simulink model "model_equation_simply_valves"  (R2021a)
settings: Solver=FixedStepAuto  StartTime=0.0  StopTime=10.0  FixedStep=Ts  RelTol=1e-3
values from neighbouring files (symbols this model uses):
  acc_bm = 1e-2    (= 0.01)    [params.m]
  acc_C = -1/g    (= -0.101936799185)    [params.m]
  acc_enable = 1    [params.m]
  acc_km = 1e-1    (= 0.1)    [params.m]
  acc_noise_var = 1e-2    (= 0.01)    [params.m]
  air_leak = 1    [ensemble_generate_from_model.m]    (also in params.m = 0)
  B_hs = 1e2    (= 100)    [params.m]
  b_large_bot = 1400    [params.m]
  b_large_up = 1400    [params.m]
  b_small_bot = 1082.6    [params.m]    (also in load_fault_code_params.m)
  b_small_up = 1543.1    [params.m]    (also in load_fault_code_params.m)
  bot_damp_start = 0.01054    [params.m]
  C_1 = sqrt(gamma/R*(2/(gamma+1))^((gamma+1)/(gamma-1)))    [params.m]
  C_2 = sqrt((2*gamma)/(R*(gamma-1)))    [params.m]
  C_A_in = 6.8608e-07    [params.m]    (also in load_fault_code_params.m)
  C_A_out = 5.2299e-07    [params.m]    (also in load_fault_code_params.m)
  C_B_in = 1.8721e-07    [params.m]    (also in load_fault_code_params.m)
  C_B_out = 9.8141e-07    [params.m]    (also in load_fault_code_params.m)
  C_leak = 1e-15    [params.m]
  counter_bits = 32    [params.m]
  cycle = 0    [params.m]    (also in ensemble_process.m = data.Cycle{1,1}.Data)
  F_c = 0    [params.m]
  F_df = 0    [params.m]
  F_sf = 0    [params.m]
  flow_C = flow_enable/flow_C_ratio/conv_SI    (= 59999.988)    [params.m]
  flow_C_ratio = dm_max/U_f_max    (= 1)    [params.m]
  flow_noise_var = 1e-6    (= 1e-06)    [params.m]
  flow_noise_var_con = 1e-6    (= 1e-06)    [params.m]
  flow_offset_con = 0    [params.m]
  flow_offset_ex = 0    [params.m]
  g = 9.81    [params.m]    (also in Conversion_Acc.m)
  gamma = 1.4    [params.m]
  gn = 0    [params.m]
  gp = 0.19382    [params.m]
  id = 0    [params.m]
  K_hs = 1e7    (= 10000000)    [params.m]
  k_small_bot = 0    [params.m]
  k_small_up = 0    [params.m]
  L = 0.2    [params.m]    (also in hammerstein_wiener_model_estimation.m = NaN(N,nk))
  LargeDamper_bottom = member.LargeDamper_bottom{1,1}.Variables    [identification_faultcode.m]    (also in params.m = 0; config_print.m; models_compire.m)
  LargeDamper_upper = member.LargeDamper_upper{1,1}.Variables    [identification_faultcode.m]    (also in params.m = 0; config_print.m; models_compire.m)
  M = 6.7798462575453    (= 6.77984625755)    [params.m]
  M_L = member.("Settings.Load"){1,1}{1,1}    [identification_faultcode.m]    (also in params.m = 6.25; config_print.m; models_compire.m)
  P_0 = 101325    [params.m]
  p_A0 = P_0    (= 101325)    [params.m]
  p_B0 = P_s    (= 600000)    [params.m]
  P_cr = 0.20105    [params.m]    (also in load_fault_code_params.m)
  P_cr_ref = P_cr    (= 0.528281787717)    [params.m]
  P_s = 6e5    (= 600000)    [params.m]
  prox_bot_band = 4e-4    (= 0.0004)    [params.m]
  prox_up_band = 0.1925    [params.m]
  R = 287.1    [params.m]
  resolution = 7.8125e-6    (= 7.8125e-06)    [params.m]    (also in filtering.m; Conversion_Enc.m; pokus.m)
  S_0 = S_A-S_B    (= 5.02654824574e-05)    [params.m]
  S_A = (pi*d_A^2)/4    (= 0.000314159265359)    [params.m]
  S_B = S_A-(pi*d_S^2)/4    (= 0.000263893782902)    [params.m]
  sg_C = Us/F_max    (= 0.005)    [params.m]
  sg_enable = 1    [params.m]
  sg_noise_var = 1e-1    (= 0.1)    [params.m]
  SmallDamper_bottom = member.SmallDamper_bottom{1,1}.Variables    [identification_faultcode.m]    (also in params.m = 6; config_print.m; models_compire.m)
  SmallDamper_upper = member.SmallDamper_upper{1,1}.Variables    [identification_faultcode.m]    (also in params.m = 4; config_print.m; models_compire.m)
  spool_dynamic = 0.02116    [params.m]
  spool_valve_time_delay = 0.01    [params.m]
  T = 281.7    [params.m]    (also in identification_nn.m = cell2mat(T); nn_using.m = tonndata(mimo_T,false,false); nn.m = T(3:end); data_parser.m = T(3:end))
  threshold = 2^(counter_bits - 1)    (= 2147483648)    [params.m]
  Ts = 1/Freq    (= 0.001)    [params.m]    (also in hammerstein_wiener_model_estimation.m; extract_signals_from_member.m; models_compire.m)
  up_damp_start = 0.18123    [params.m]
  V_0A = S_A*0.015    (= 4.71238898038e-06)    [params.m]
  V_0B = S_B*0.015    (= 3.95840674352e-06)    [params.m]
libraries: eeQuadratureDecoder x1

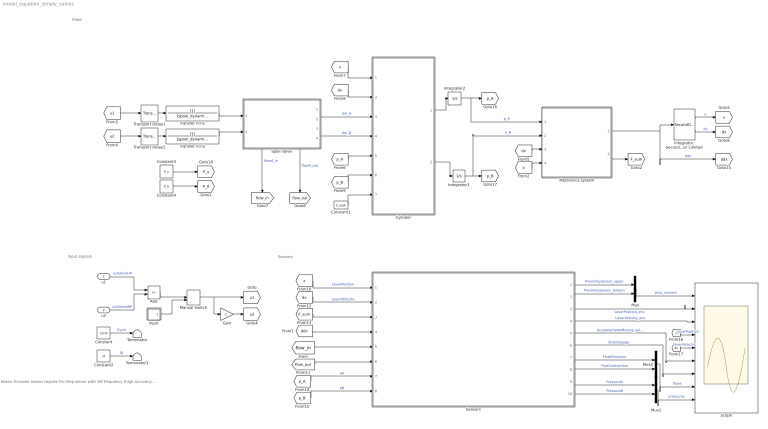
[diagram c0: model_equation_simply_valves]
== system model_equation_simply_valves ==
  note: Sensors
  note: Notes: Encoder sensor require Fix-Step solver with 1M frequency (high accuracy of sensor). For faster-simulation Ts = 1e-3.
  note: Plant
  note: Input signals
  u1 : Inport
  u2 : Inport  Port=2
  Add : Sum  Inputs=-+
  Constant : Constant  Value=cycle  OutDataTypeStr=double
  Constant1 : Constant  Value=C_leak
  Constant2 : Constant  Value=id  OutDataTypeStr=double
  Constant3 : Constant  Value=P_s
  Constant4 : Constant  Value=P_0
  Cylinder : MATLAB Function  TreatAsAtomicUnit=on
  Gain : Gain  Gain=-1
  "Integrator, Second-Order Limited" : SecondOrderIntegrator  ICX=x0  UpperLimitX=gp  LowerLimitX=gn
  Integrator2 : Integrator  InitialCondition=p_A0
  Integrator3 : Integrator  InitialCondition=p_B0
  Manual Switch : ManualSwitch  CurrentSetting=0
  Mechanica system : MATLAB Function  TreatAsAtomicUnit=on
  Mux : Mux  Inputs=2
  Mux1 : Mux  Inputs=2
  Mux2 : Mux  Inputs=2
  Scope : Scope  NumInputPorts=9
  Sensors : Subsystem
  Spoll valve : Subsystem
  Terminator : Terminator
  Terminator1 : Terminator
  Transfer Fcn1 : TransferFcn  Denominator=[spool_dynamic 1]
  Transfer Fcn2 : TransferFcn  Denominator=[spool_dynamic 1]
  Transport Delay1 : TransportDelay  DelayTime=spool_valve_time_delay
  Transport Delay2 : TransportDelay  DelayTime=spool_valve_time_delay
  input : Subsystem
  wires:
  Sensors/3(encoder_LeverPosition) -> Scope/2  "LeverPosition_enc"
  [ddx] -> Sensors/4(ddx)
  input/1(Out1) -> Manual Switch/2
  Sensors/8(FlowContraction) -> Mux2/2  "FlowContraction"
  Mechanica system/1(ddx) -> [ddx], "Integrator, Second-Order Limited"/1  "ddx"
  Constant3/1 -> [P_s]
  [dx] -> Sensors/2(LeverVelocity)  "LeverVelocity"
  [p_B] -> Sensors/8(pB)  "pB"
  u1/1 -> Add/1  "outValveHP"
  Integrator2/1 -> [p_A], Mechanica system/1(p_A)  "p_A"
  Add/1 -> Manual Switch/1
  Mux2/1 -> Scope/8  "flows"
  Transport Delay2/1 -> Transfer Fcn2/1
  Manual Switch/1 -> Gain/1, [u1]
  Sensors/1(ProximitySensor_upper) -> Mux/1  "ProximitySensor_upper"
  "Integrator, Second-Order Limited"/2 -> [dx]  "dx"
  Transfer Fcn1/1 -> Spoll valve/1(u_A)
  Spoll valve/4(flow_out) -> [flow_out]  "flowA_out"
  [flow_in] -> Sensors/5(dm_A_in)
  Transfer Fcn2/1 -> Spoll valve/2(u_B1)
  [F_sum] -> Sensors/3(F)
  [dx] -> Mechanica system/3(dx)
  [u1] -> Transport Delay1/1
  Sensors/2(ProximitySensor_bottom) -> Mux/2  "ProximitySensor_bottom"
  [p_B] -> Cylinder/6(p_B)
  Sensors/4(encoder_LeverVelocity) -> Scope/3  "LeverVelocity_enc"
  Spoll valve/1(dm_A) -> Cylinder/3(dm_A)  "dm_A"
  Spoll valve/3(flow_in) -> [flow_in]  "flowA_in"
  Sensors/7(FlowExtrusion) -> Mux2/1  "FlowExtrusion"
  [x] -> Cylinder/1(x)
  u2/1 -> Add/2  "outValveWP"
  [p_A] -> Cylinder/5(p_A)
  [dx] -> Scope/5  "LeverVelocity"
  [x] -> Sensors/1(LeverPosition)  "LeverPosition"
  [p_A] -> Sensors/7(pA)  "pA"
  Sensors/9(PressureA) -> Mux1/1  "PressureA"
  Spoll valve/2(dm_B) -> Cylinder/4(dm_B)  "dm_B"
  Transport Delay1/1 -> Transfer Fcn1/1
  "Integrator, Second-Order Limited"/1 -> [x]  "x"
  Sensors/5(AccelerometerMoving axisZ) -> Scope/6  "AccelerometerMoving_axisZ"
  [dx] -> Cylinder/2(dx)
  Mechanica system/2(F_sum_strain) -> [F_sum]
  Mux/1 -> Scope/1  "prox_sensors"
  [flow_out] -> Sensors/6(dm_A_out)
  Sensors/6(StrainGauge) -> Scope/7  "StrainGauge"
  Mux1/1 -> Scope/9  "pressures"
  Gain/1 -> [u2]
  [x] -> Scope/4  "LeverPosition"
  [u2] -> Transport Delay2/1
  Constant/1 -> Terminator/1  "Cycle"
  Sensors/10(PressureB) -> Mux1/2  "PressureB"
  Cylinder/1(dp_A) -> Integrator2/1
  Constant1/1 -> Cylinder/7(C_leak)
  [x] -> Mechanica system/4(x)
  Constant4/1 -> [P_0]
  Integrator3/1 -> Mechanica system/2(p_B), [p_B]  "p_B"
  Cylinder/2(dp_B) -> Integrator3/1
  Constant2/1 -> Terminator1/1  "ID"

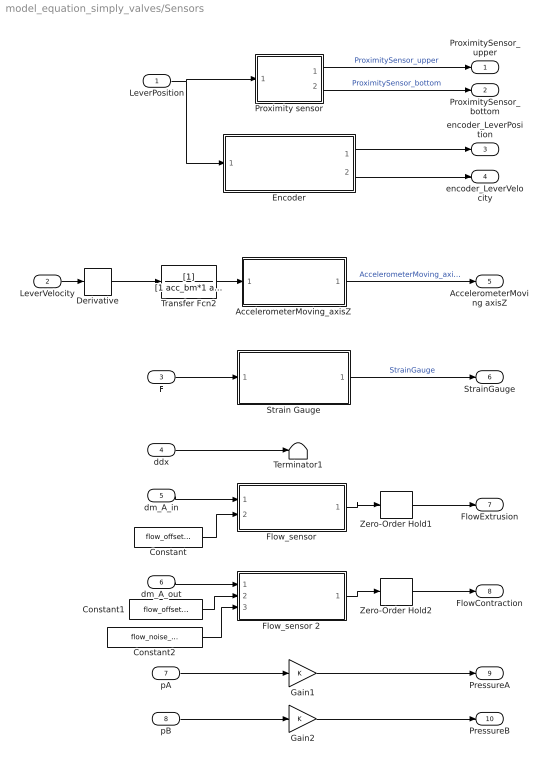
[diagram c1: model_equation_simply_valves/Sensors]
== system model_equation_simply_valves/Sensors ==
  LeverPosition : Inport
  LeverVelocity : Inport  Port=2
  F : Inport  Port=3
  ddx : Inport  Port=4
  dm_A_in : Inport  Port=5
  dm_A_out : Inport  Port=6
  pA : Inport  Port=7
  pB : Inport  Port=8
  AccelerometerMoving_axisZ : MATLAB Function  TreatAsAtomicUnit=on
  Constant : Constant  Value=flow_offset_ex
  Constant1 : Constant  Value=flow_offset_con
  Constant2 : Constant  Value=flow_noise_var_con
  Derivative : Derivative
  Encoder : Subsystem
  Flow_sensor : MATLAB Function  TreatAsAtomicUnit=on
  Flow_sensor 2 : MATLAB Function  TreatAsAtomicUnit=on
  Gain1 : Gain
  Gain2 : Gain
  Proximity sensor : MATLAB Function  TreatAsAtomicUnit=on
  Strain Gauge : MATLAB Function  TreatAsAtomicUnit=on
  Terminator1 : Terminator
  Transfer Fcn2 : TransferFcn  Denominator=[1 acc_bm*1 acc_km*1]
  Zero-Order Hold1 : ZeroOrderHold  SampleTime=Ts
  Zero-Order Hold2 : ZeroOrderHold  SampleTime=Ts
  ProximitySensor_upper : Outport
  ProximitySensor_bottom : Outport  Port=2
  encoder_LeverPosition : Outport  Port=3
  encoder_LeverVelocity : Outport  Port=4
  AccelerometerMoving axisZ : Outport  Port=5
  StrainGauge : Outport  Port=6
  FlowExtrusion : Outport  Port=7
  FlowContraction : Outport  Port=8
  PressureA : Outport  Port=9
  PressureB : Outport  Port=10
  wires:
  F/1 -> Strain Gauge/1(F)
  dm_A_out/1 -> Flow_sensor 2/1(dm_A)
  pB/1 -> Gain2/1
  Flow_sensor/1(dm_A_sensor) -> Zero-Order Hold1/1
  ddx/1 -> Terminator1/1
  AccelerometerMoving_axisZ/1(acc_measured) -> AccelerometerMoving axisZ/1  "AccelerometerMoving_axisZ"
  Encoder/1(encoder_LeverPosition) -> encoder_LeverPosition/1
  Gain2/1 -> PressureB/1
  Proximity sensor/1(up) -> ProximitySensor_upper/1  "ProximitySensor_upper"
  LeverVelocity/1 -> Derivative/1
  Strain Gauge/1(F_measured) -> StrainGauge/1  "StrainGauge"
  Flow_sensor 2/1(dm_A_sensor) -> Zero-Order Hold2/1
  Proximity sensor/2(bot) -> ProximitySensor_bottom/1  "ProximitySensor_bottom"
  Zero-Order Hold2/1 -> FlowContraction/1
  pA/1 -> Gain1/1
  dm_A_in/1 -> Flow_sensor/1(dm_A)
  Zero-Order Hold1/1 -> FlowExtrusion/1
  LeverPosition/1 -> Encoder/1(x), Proximity sensor/1(x)
  Gain1/1 -> PressureA/1
  Encoder/2(encoder_LeverVelocity) -> encoder_LeverVelocity/1
  Constant/1 -> Flow_sensor/2(flow_offset)
  Constant1/1 -> Flow_sensor 2/2(flow_offset)
  Constant2/1 -> Flow_sensor 2/3(flow_noise_var)
  Derivative/1 -> Transfer Fcn2/1
  Transfer Fcn2/1 -> AccelerometerMoving_axisZ/1(ddx)

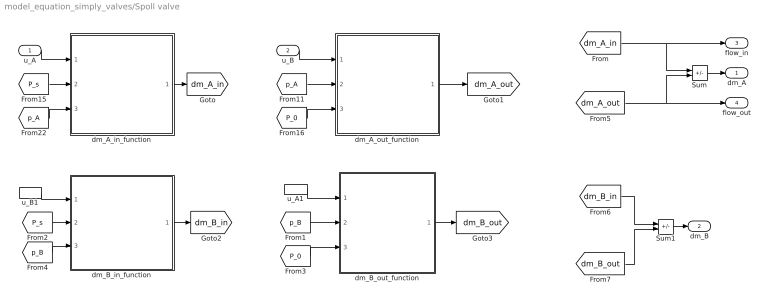
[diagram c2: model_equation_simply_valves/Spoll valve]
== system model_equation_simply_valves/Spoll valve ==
  u_A : Inport
  u_B : Inport  Port=2
  Sum : Sum  Inputs=+-
  Sum1 : Sum  Inputs=+-
  dm_A_in_function : MATLAB Function  TreatAsAtomicUnit=on
  dm_A_out_function : MATLAB Function  TreatAsAtomicUnit=on
  dm_B_in_function : MATLAB Function  TreatAsAtomicUnit=on
  dm_B_out_function : MATLAB Function  TreatAsAtomicUnit=on
  u_A1 : InportShadow
  u_B1 : InportShadow  Port=2
  dm_A : Outport
  dm_B : Outport  Port=2
  flow_in : Outport  Port=3
  flow_out : Outport  Port=4
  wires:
  [P_s] -> dm_A_in_function/2(P_u)
  [p_A] -> dm_A_in_function/3(P_d)
  dm_A_in_function/1(dm) -> [dm_A_in]
  dm_A_out_function/1(dm) -> [dm_A_out]
  [p_A] -> dm_A_out_function/2(P_u)
  [P_0] -> dm_A_out_function/3(P_d)
  u_A/1 -> dm_A_in_function/1(u)
  u_B/1 -> dm_A_out_function/1(u)
  u_B1/1 -> dm_B_in_function/1(u)
  [P_0] -> dm_B_out_function/3(P_d)
  [p_B] -> dm_B_out_function/2(P_u)
  [p_B] -> dm_B_in_function/3(P_d)
  [P_s] -> dm_B_in_function/2(P_u)
  u_A1/1 -> dm_B_out_function/1(u)
  dm_B_in_function/1(dm) -> [dm_B_in]
  dm_B_out_function/1(dm) -> [dm_B_out]
  Sum/1 -> dm_A/1
  Sum1/1 -> dm_B/1
  [dm_A_in] -> flow_in/1, Sum/1
  [dm_A_out] -> flow_out/1, Sum/2
  [dm_B_in] -> Sum1/1
  [dm_B_out] -> Sum1/2

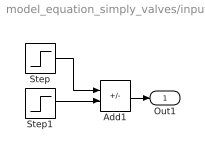
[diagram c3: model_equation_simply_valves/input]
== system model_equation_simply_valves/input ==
  Add1 : Sum  Inputs=+-
  Step : Step  Before=-1  SampleTime=0
  Step1 : Step  Time=6  After=2  SampleTime=0
  Out1 : Outport
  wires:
  Step/1 -> Add1/1
  Step1/1 -> Add1/2
  Add1/1 -> Out1/1

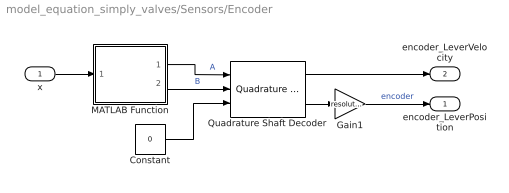
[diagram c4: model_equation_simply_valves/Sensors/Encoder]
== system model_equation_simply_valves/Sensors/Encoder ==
  x : Inport
  Constant : Constant  Value=0
  Gain1 : Gain  Gain=resolution*2
  MATLAB Function : MATLAB Function  TreatAsAtomicUnit=on
  Quadrature Shaft Decoder : eeQuadratureDecoder/Quadrature Shaft Decoder  NPulse=4  Ts=Ts
  encoder_LeverPosition : Outport
  encoder_LeverVelocity : Outport  Port=2
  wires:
  x/1 -> MATLAB Function/1(x)
  MATLAB Function/2(B) -> Quadrature Shaft Decoder/2  "B"
  Quadrature Shaft Decoder/2 -> Gain1/1
  Gain1/1 -> encoder_LeverPosition/1  "encoder"
  MATLAB Function/1(A) -> Quadrature Shaft Decoder/1  "A"
  Constant/1 -> Quadrature Shaft Decoder/3
  Quadrature Shaft Decoder/1 -> encoder_LeverVelocity/1

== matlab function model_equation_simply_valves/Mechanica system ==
function [ddx, F_sum_strain] = fcn(p_A,p_B,dx,x,S_A,S_B,M,M_L,P_0,S_0,g, ...
    up_damp_start,bot_damp_start,b_small_up,k_small_up,b_small_bot,k_small_bot,SmallDamper_bottom,SmallDamper_upper, ...
    K_hs,B_hs,gp,gn,b_large_bot, b_large_up, LargeDamper_bottom, LargeDamper_upper, F_sf, F_df, F_c)



% % Hard Stop
if 1
up_force = K_hs*(x-gp) + B_hs*dx*ge(dx,0);
bot_force = K_hs*(x-gn) + B_hs*dx*le(dx,0);
% up_force = K_hs*(x-gp) + B_hs*dx*abs(x-gp);
% bot_force = K_hs*(x-gn) + B_hs*dx*abs(x-gn);

% Dead zone calculating Hard Stop
if x >= gp
    F_hs = up_force;
elseif x > gn
    F_hs = 0;
else
    F_hs = bot_force;
end

else
F_hs = 0;
end
% Pneumatic equation
F_pneum = p_A*S_A - p_B*S_B - P_0*S_0;

% Viscous Force
% beta1 = beta + 0.001;
% F_f = dx*beta1;
% F_f = sign(dx) * (1 * abs(dx) + 1);
if dx == 0
    F_sd = F_sf;
else
    F_sd = 0;
end
F_f = F_df*dx + F_c*sign(dx) + F_sd;



% Dead zone calculating Small Dampers
up_force = k_small_up*(x-up_damp_start) + SmallDamper_upper*b_small_up*dx*ge(dx,0);
bot_force = k_small_bot*(x-bot_damp_start) + SmallDamper_bottom*b_small_bot*dx*le(dx,0);

if x >= up_damp_start
    F_damp_small = up_force;
elseif x > bot_damp_start
    F_damp_small = 0;
else
    F_damp_small = bot_force;
end


% Dead zone calculating Small Dampers
up_force =  LargeDamper_upper*b_large_up*dx*ge(dx,0);
bot_force =  LargeDamper_bottom*b_large_bot*dx*le(dx,0);

if x >= up_damp_start
    F_damp_large = up_force;
elseif x > bot_damp_start
    F_damp_large = 0;
else
    F_damp_large = bot_force;
end

F_damp = F_damp_small + F_damp_large;

% Gravity
F_g = (M + M_L)*g;

F_sum_strain = F_pneum - F_g;
F_sum = (F_pneum - F_f - F_hs - F_g - F_damp);
% Full mechincal equation
ddx = 1/(M+M_L)*F_sum;
end

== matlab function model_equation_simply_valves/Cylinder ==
function [dp_A,dp_B]= fcn(x,dx,dm_A,dm_B,p_A,p_B,gamma,V_0A,V_0B,S_A,S_B,R,T,L,P_cr_ref,C_2,C_1,air_leak,P_0, C_leak)

V_A = V_0A + S_A*x;
dV_A = dx * S_A;

V_B = V_0B + S_B*(L-x);
dV_B = - dx * S_B;

% Air leak on chamber B model

if air_leak  
    P_d = P_0;
    P_u = p_B;
    P_ratio = P_d/P_u;
    if P_ratio <= P_cr_ref && P_ratio >= 0
        dm_leak = C_leak*C_1*P_u/sqrt(T);
    elseif P_ratio > P_cr_ref && P_ratio <= 1
        dm_leak = C_leak*C_2*P_u/sqrt(T)*P_ratio^(1/gamma)*sqrt(1-P_ratio^((gamma-1)/gamma));
        %dm = u*C_B_in*P_u*sqrt(1-((P_ratio - P_cr)/(1-P_cr))^2);
    else
       %dm_leak = -C_leak*C_2*P_d/sqrt(T)*(1/P_ratio)^(1/gamma)*sqrt(1-(1/P_ratio)^((gamma-1)/gamma));
        dm_leak = 0;
    end
else
    dm_leak = 0;
end



dp_A = dm_A*gamma*R*T/V_A - p_A*gamma*dV_A/V_A;
dp_B = (dm_B-dm_leak)*gamma*R*T/V_B - p_B*gamma*dV_B/V_B;
dm_leak = dm_B - dm_leak;

end

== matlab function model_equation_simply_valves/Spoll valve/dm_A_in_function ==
function dm = fcn(u, P_u, P_d, C_A_in, C_1, C_2, P_cr, T, gamma)
if u > 0    
    P_ratio = P_d/P_u;
    if P_ratio <= P_cr && P_ratio >= 0
        dm = u*C_A_in*C_1*P_u/sqrt(T);
    elseif P_ratio > P_cr && P_ratio <= 1
        dm = u*C_A_in*C_2*P_u/sqrt(T)*P_ratio^(1/gamma)*sqrt(1-P_ratio^((gamma-1)/gamma));
        %dm = u*C_A_in*P_u*sqrt(1-((P_ratio - P_cr)/(1-P_cr))^2);
    else
        %dm = -u*C_A_in*C_2*P_d/sqrt(T)*(1/P_ratio)^(1/gamma)*sqrt(1-(1/P_ratio)^((gamma-1)/gamma));
        dm = 0;
    end
else
    dm = 0;
end

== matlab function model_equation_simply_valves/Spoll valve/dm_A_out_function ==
function dm = fcn(u, P_u, P_d, C_A_out, C_1, P_cr, C_2, T, gamma)
if u > 0    
    P_ratio = P_d/P_u;
    if P_ratio <= P_cr && P_ratio >= 0
        dm = u*C_A_out*C_1*P_u/sqrt(T);
    elseif P_ratio > P_cr && P_ratio <= 1
        dm = u*C_A_out*C_2*P_u/sqrt(T)*P_ratio^(1/gamma)*sqrt(1-P_ratio^((gamma-1)/gamma));
        %dm = u*C_A_out*P_u*sqrt(1-((P_ratio - P_cr)/(1-P_cr))^2);

    else
        %dm = -u*C_A_out*C_2*P_d/sqrt(T)*(1/P_ratio)^(1/gamma)*sqrt(1-(1/P_ratio)^((gamma-1)/gamma));
        dm = 0;
    end
else
    dm = 0;
end

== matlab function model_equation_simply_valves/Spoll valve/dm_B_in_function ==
function dm = fcn(u, P_u, P_d, P_cr, C_B_in, C_1, C_2, T, gamma)
if u > 0    
    P_ratio = P_d/P_u;
    if P_ratio <= P_cr && P_ratio >= 0
        dm = u*C_B_in*C_1*P_u/sqrt(T);
    elseif P_ratio > P_cr && P_ratio <= 1
        dm = u*C_B_in*C_2*P_u/sqrt(T)*P_ratio^(1/gamma)*sqrt(1-P_ratio^((gamma-1)/gamma));
        %dm = u*C_B_in*P_u*sqrt(1-((P_ratio - P_cr)/(1-P_cr))^2);

    else
        %dm = -u*C_B_in*C_2*P_d/sqrt(T)*(1/P_ratio)^(1/gamma)*sqrt(1-(1/P_ratio)^((gamma-1)/gamma));
        dm = 0;
    end
else
    dm = 0;
end

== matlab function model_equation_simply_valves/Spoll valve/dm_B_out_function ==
function dm = fcn(u, P_u, P_d, P_cr, C_B_out, C_1, C_2, T, gamma)
if u > 0    
    P_ratio = P_d/P_u;
    if P_ratio <= P_cr && P_ratio >= 0
        dm = u*C_B_out*C_1*P_u/sqrt(T);
    elseif P_ratio > P_cr && P_ratio <= 1
        dm = u*C_B_out*C_2*P_u/sqrt(T)*P_ratio^(1/gamma)*sqrt(1-P_ratio^((gamma-1)/gamma));
        %dm = u*C_B_out*P_u*sqrt(1-((P_ratio - P_cr)/(1-P_cr))^2);

    else
        %dm = -u*C_B_out*C_2*P_d/sqrt(T)*(1/P_ratio)^(1/gamma)*sqrt(1-(1/P_ratio)^((gamma-1)/gamma));
        dm = 0;
    end
else
    dm = 0;
end

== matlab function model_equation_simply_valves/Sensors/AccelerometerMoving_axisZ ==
function acc_measured = fcn(ddx, acc_noise_var, acc_enable, acc_C)

ZeroOffset = 2.5; % V
Sensetivity = 333; %mv/g

acc = acc_enable * acc_C * ddx + 1;

U_raw = acc*Sensetivity/1000 + ZeroOffset;
U_raw = U_raw + acc_noise_var*(2*rand()-1);

acc_measured =  acc_enable*((U_raw - ZeroOffset)*1000/Sensetivity);
end

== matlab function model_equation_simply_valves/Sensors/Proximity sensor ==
function [up,bot]= fcn(x, prox_up_band, prox_bot_band)
if x >= prox_up_band
    up = 1; bot = 0;
elseif x <= prox_bot_band
    bot = 1; up = 0;
else
    bot = 0;
    up = 0;
end

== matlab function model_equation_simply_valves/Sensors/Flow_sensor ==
function dm_A_sensor = fcn(dm_A, flow_C, flow_C_ratio, flow_noise_var, flow_offset)
dm_A_sensor = flow_C*(flow_C_ratio*dm_A + flow_noise_var*(2*rand()-1)) + flow_offset;
end

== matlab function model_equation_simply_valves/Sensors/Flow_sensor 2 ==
function dm_A_sensor = fcn(dm_A, flow_C, flow_C_ratio, flow_offset, flow_noise_var)
dm_A_sensor = flow_C*(flow_C_ratio*dm_A + flow_noise_var*(2*rand()-1)) + flow_offset;

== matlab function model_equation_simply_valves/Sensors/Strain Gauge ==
function F_measured = fcn(F,sg_enable, sg_noise_var, sg_C)
U = sg_enable*(sg_C*F + sg_noise_var*(2*rand()-1));
F_measured = U*1/sg_C;
end

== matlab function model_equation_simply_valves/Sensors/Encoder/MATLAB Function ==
function [A, B]= fcn(x, resolution, counter_bits, threshold)
period = 4*resolution;
a = mod(x, period);
b = mod(x-resolution, period);
if 0 < a && a < period/2
    A = 1;
elseif period/2 < a && a < period
    A = 0;
else
    A = 0;
end

if 0 < b && b < period/2
    B = 1;
elseif period/2 < b && b < period
    B = 0;
else 
    B = 0;
end
